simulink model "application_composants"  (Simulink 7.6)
settings: Solver=ode14x  StartTime=0.0  StopTime=N  RelTol=1e-3
InitFcn:
  | clc, clear all, close all
  | N=0.02;
StopFcn:
  | close all
  | load vitesse_position.mat
  | plotyy(x(1,:),x(2,:),x(1,:),x(3,:))
  | grid
  | title('Position et vitesse angulaires')
  | delete *.mat
undefined symbols (not defined in the file or in its folder): sigbuilder_block
libraries: fl_lib x7, nesl_utility x4, AppliMechanical_lib x2, AppliElectrical_lib x1

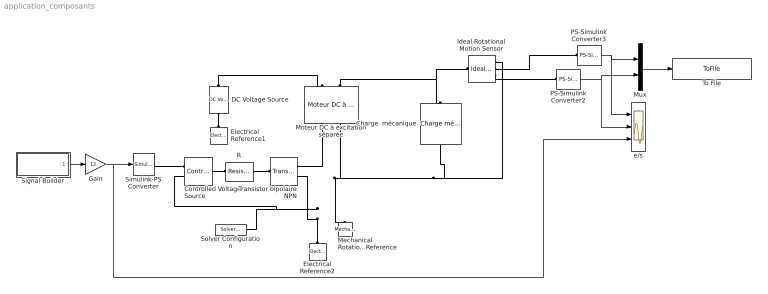
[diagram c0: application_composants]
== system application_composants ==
  Charge  mécanique : AppliMechanical_lib/Charge mécanique  DialogController=NetworkEngine.DynNeDlgSource  SystemSampleTime=-1  k=100 N*m/rad  J=2 kg*m^2  fr=500 N*m/(rad/s)  alpha_Log=off  t_Log=off  w_Log=off  LocalVarNames=|alpha|t|w  LocalVarDescs=|alpha|t|w  LocalVarLogging=[0 0 0]
  Controlled Voltage Source : fl_lib/Electrical/Electrical Sources/Controlled Voltage Source  DialogController=NetworkEngine.DynNeDlgSource  SystemSampleTime=-1  i_Log=off  v_Log=off  LocalVarNames=|i|v  LocalVarDescs=|i|v  LocalVarLogging=[0 0]
  DC Voltage Source : fl_lib/Electrical/Electrical Sources/DC Voltage Source  DialogController=NetworkEngine.DynNeDlgSource  SystemSampleTime=-1  v0=12 V  i_Log=off  v_Log=off  LocalVarNames=|i|v  LocalVarDescs=|i|v  LocalVarLogging=[0 0]
  Electrical Reference1 : fl_lib/Electrical/Electrical Elements/Electrical Reference  DialogController=NetworkEngine.DynNeDlgSource  SystemSampleTime=-1  i_Log=off  LocalVarNames=|i  LocalVarDescs=|i  LocalVarLogging=[]
  Electrical Reference2 : fl_lib/Electrical/Electrical Elements/Electrical Reference  DialogController=NetworkEngine.DynNeDlgSource  SystemSampleTime=-1  i_Log=off  LocalVarNames=|i  LocalVarDescs=|i  LocalVarLogging=[]
  Gain : Gain  Gain=12
  Ideal Rotational Motion Sensor : fl_lib/Mechanical/Mechanical Sensors/Ideal Rotational Motion Sensor  DialogController=NetworkEngine.DynNeDlgSource  SystemSampleTime=-1  offset=0 rad  w_Log=off  t_Log=off  phi_Log=off  LocalVarNames=|w|t|phi  LocalVarDescs=|w|t|phi  LocalVarLogging=[0 0 0]
  Mechanical Rotational Reference : fl_lib/Mechanical/Rotational Elements/Mechanical Rotational Reference  DialogController=NetworkEngine.DynNeDlgSource  SystemSampleTime=-1  t_Log=off  LocalVarNames=|t  LocalVarDescs=|t  LocalVarLogging=[]
  Moteur DC à excitation séparée : AppliMechanical_lib/Moteur DC à excitation séparée  DialogController=NetworkEngine.DynNeDlgSource  SystemSampleTime=-1  K=0.1 N*m/A  Ri=4.9 Ohm  Li=1e-5 H  fr=0.02 N*m/(rad/s)  J=1e-5 kg*m^2  w_Log=off  i_Log=off  v_Log=off  t_Log=off  LocalVarNames=|w|i|v|t  LocalVarDescs=|w|i|v|t  LocalVarLogging=[0 0 0 0]
  Mux : Mux  Inputs=2
  PS-Simulink Converter2 : nesl_utility/PS-Simulink Converter  DialogController=NetworkEngine.DynNeUtilDlgSource  SystemSampleTime=-1  PhysicalDomain=network_engine_domain  LeftPortType=input  RightPortType=output  SubClassName=ps_output  Unit=1  AffineConversion=off
  PS-Simulink Converter3 : nesl_utility/PS-Simulink Converter  DialogController=NetworkEngine.DynNeUtilDlgSource  SystemSampleTime=-1  PhysicalDomain=network_engine_domain  LeftPortType=input  RightPortType=output  SubClassName=ps_output  Unit=1  AffineConversion=off
  R : fl_lib/Electrical/Electrical Elements/Resistor  DialogController=NetworkEngine.DynNeDlgSource  SystemSampleTime=-1  R=2.2 kOhm  i_Log=off  v_Log=off  LocalVarNames=|i|v  LocalVarDescs=|i|v  LocalVarLogging=[0 0]
  Signal Builder : Subsystem  Tag=STV Subsys  LoadFcn=sigbuilder_block('load');  StartFcn=sigbuilder_block('start');  StopFcn=sigbuilder_block('stop');  ClipboardFcn=sigbuilder_block('clipboard');
  Simulink-PS Converter : nesl_utility/Simulink-PS Converter  DialogController=NetworkEngine.DynNeUtilDlgSource  SystemSampleTime=-1  PhysicalDomain=network_engine_domain  LeftPortType=input  RightPortType=output  SubClassName=ps_input  Unit=1  AffineConversion=off  InputFilterTimeConstant=.001  UdotUserProvided=0
  Solver Configuration : nesl_utility/Solver Configuration  DialogController=NetworkEngine.DynNeUtilDlgSource  SystemSampleTime=-1  PhysicalDomain=network_engine_domain  LeftPortType=input  RightPortType=generic  SubClassName=solver  Accelerate=off  Profile=off  ResidualTolerance=1e-9  MaxNonlinIter=3  MaxModeIter=2  DoFixedCost=off  UseLocalSampling=off  DoDC=off  LinearAlgebra=Sparse  LocalSolverSampleTime=.001  LocalSolverChoice=NE_BACKWARD_EULER_ADVANCER  UseLocalSolver=off
  To File : ToFile  Filename=vitesse_position  MatrixName=x
  Transistor bipolaire NPN : AppliElectrical_lib/Transistor bipolaire NPN  DialogController=NetworkEngine.DynNeDlgSource  SystemSampleTime=-1  s=1e-6 1/Ohm  h21=200  h12=1e-4  h11=1000 Ohm  Ib_Log=off  Vbe_Log=off  Ic_Log=off  Vce_Log=off  LocalVarNames=|Ib|Vbe|Ic|Vce  LocalVarDescs=|courant d'entrée du transistor|tension, Base-Emetteur|courant Collecteur-Emetteur|tension Collecteur-Emetteur  LocalVarLogging=[0 0 0 0]
  e/s : Scope  NumInputPorts=3
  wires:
  Signal Builder/1(Signal 2) -> Gain/1
  Gain/1 -> Simulink-PS Converter/1, e/s/3
  PS-Simulink Converter2/1 -> Mux/2, e/s/2
  PS-Simulink Converter3/1 -> Mux/1, e/s/1
  Mux/1 -> To File/1
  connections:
  Ideal Rotational Motion Sensor/RConn1 -- Moteur DC à excitation séparée/RConn2 -- Mechanical Rotational Reference/LConn1 -- Charge  mécanique/RConn1
  Moteur DC à excitation séparée/LConn2 -- Charge  mécanique/LConn1 -- Ideal Rotational Motion Sensor/LConn1
  Ideal Rotational Motion Sensor/RConn2 -- PS-Simulink Converter3/LConn1
  Ideal Rotational Motion Sensor/RConn3 -- PS-Simulink Converter2/LConn1
  Moteur DC à excitation séparée/RConn1 -- Transistor bipolaire NPN/RConn1
  Electrical Reference2/LConn1 -- Transistor bipolaire NPN/RConn2 -- Controlled Voltage Source/RConn2 -- Solver Configuration/RConn1
  Simulink-PS Converter/RConn1 -- Controlled Voltage Source/RConn1
  DC Voltage Source/LConn1 -- Moteur DC à excitation séparée/LConn1
  DC Voltage Source/RConn1 -- Electrical Reference1/LConn1
  R/LConn1 -- Transistor bipolaire NPN/LConn1
  Controlled Voltage Source/LConn1 -- R/RConn1

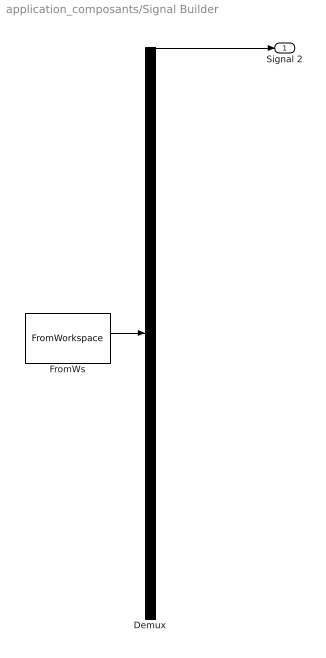
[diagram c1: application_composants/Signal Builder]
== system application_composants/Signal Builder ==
  Demux : Demux  Tag=STV Demux  Outputs=1
  FromWs : FromWorkspace  Tag=STV FromWs  VariableName=tuvar  SampleTime=0  SigBuilderData=DataTag0  VnvData=DataTag1
  Signal 2 : Outport  Tag=STV Outport
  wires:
  FromWs/1 -> Demux/1
  Demux/1 -> Signal 2/1
